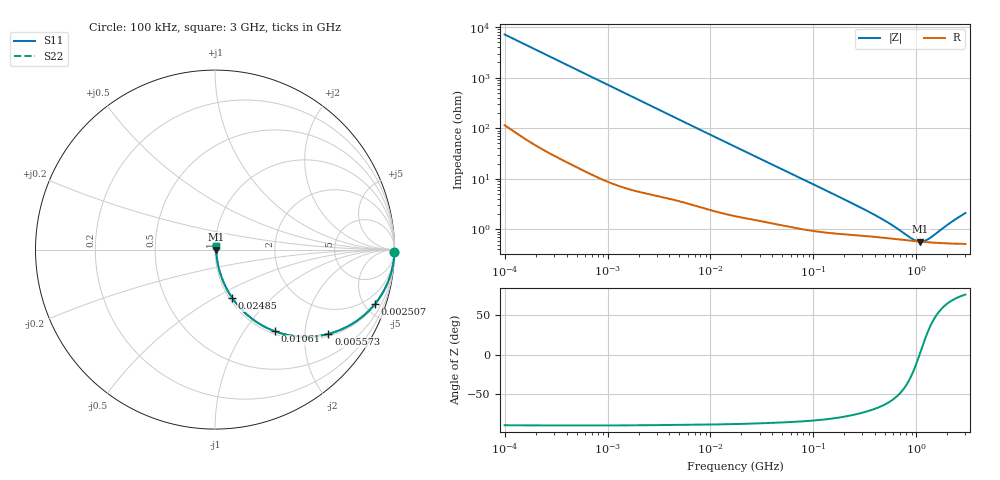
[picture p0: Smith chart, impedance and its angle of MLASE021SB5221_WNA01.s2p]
! MLASE021SB5221_WNA01  S-PARAMETER MODEL  ( Standard Model )
! Model Generated by TAIYO YUDEN Corporation (http://www.ty-top.com)
! Version 1.0
! TAIYO YUDEN Control No. 220901
! Copyright(c) 2022 TAIYO YUDEN CO.,LTD. All Rights Reserved.
! Product Description (link to TY-COMPAS)
! https://ds.yuden.co.jp/TYCOMPAS/or/detail?pn=MLASE021SB5221KWNA01&u=M
! Products Name : Multilayer Ceramic Capacitors
! Characteristics :
!  Capacitance : 220 [pF] , Rated Voltage : 16 [V] , TCC : X5R
!  Case Size : 0.25 x 0.125 / 0.0098 x 0.0049 [mm/inch] , Thickness : 0.125 / 0.0049 [mm/inch]
!  (Conditions: Temperature = 25 [degC] , DC Bias Voltage = 0 [V])
! External Node Assignments :
!  1  o---| |---o  2
! GND o---------o GND
! Frequency Range : 100kHz  -  3GHz  [ 401 STEP ]
# MHZ S RI R 50
! Freq[MHz].  S11 Real  S11 Imag  S21 Real  S21 Imag  S12 Real  S12 Imag  S22 Real  S22 Imag
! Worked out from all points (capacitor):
!   401 points, 100 kHz to 3 GHz, reference 50 ohm
!   read as one part in series: C = 222 pF near 105.3 kHz
!   lowest |Z| = 572 mohm at 1.098 GHz (marker M1)
!   series resonance near 1.076 GHz, so ESL is about 98 pH
!   S11 on the Smith chart (normalised r, x): 100 kHz: open; 2.507 MHz: 1.10, -5.81; 5.573 MHz: 1.07, -2.64; 10.61 MHz: 1.05, -1.40; 24.85 MHz: 1.03, -0.61; 3 GHz: 1.01, +0.04
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0.1  0.9996 -0.014  0.00042 0.014  0.00042 0.014  0.9996 -0.014
0.266273  0.9982 -0.0369  0.00181 0.0369  0.00181 0.0369  0.9982 -0.0369
0.562235  0.9931 -0.0772  0.0069 0.0772  0.0069 0.0772  0.9931 -0.0772
1.218153  0.9707 -0.1625  0.0293 0.1625  0.0293 0.1625  0.9707 -0.1625
2.506689  0.8901 -0.3043  0.1099 0.3043  0.1099 0.3043  0.8901 -0.3043
3.161081  0.8374 -0.3594  0.1626 0.3594  0.1626 0.3594  0.8374 -0.3594
4.197169  0.7481 -0.423  0.2519 0.423  0.2519 0.423  0.7481 -0.423
5.572849  0.6321 -0.4696  0.3679 0.4696  0.3679 0.4696  0.6321 -0.4696
7.592607  0.4868 -0.4855  0.5132 0.4855  0.5132 0.4855  0.4868 -0.4855
10.61445  0.3337 -0.4552  0.6663 0.4552  0.6663 0.4552  0.3337 -0.4552
17.7727  0.1609 -0.3466  0.8391 0.3466  0.8391 0.3466  0.1609 -0.3466
24.84619  0.0957 -0.2693  0.9043 0.2693  0.9043 0.2693  0.0957 -0.2693
47.32384  0.0365 -0.1534  0.9635 0.1534  0.9635 0.1534  0.0365 -0.1534
97.38194  0.0153 -0.0773  0.9847 0.0773  0.9847 0.0773  0.0153 -0.0773
310.5665  0.00792 -0.0235  0.9921 0.0235  0.9921 0.0235  0.00792 -0.0235
547.5153  0.00671 -0.0112  0.9933 0.0112  0.9933 0.0112  0.00671 -0.0112
916.7529  0.00588 -0.00257  0.9941 0.00257  0.9941 0.00257  0.00588 -0.00257
1097.999  0.00568 0.000328  0.9943 -0.000328  0.9943 -0.000328  0.00568 0.000328
1217.231  0.00558 0.00201  0.9944 -0.00201  0.9944 -0.00201  0.00558 0.00201
1349.411  0.00551 0.00373  0.9945 -0.00373  0.9945 -0.00373  0.00551 0.00373
2201.951  0.00538 0.0129  0.9946 -0.0129  0.9946 -0.0129  0.00538 0.0129
3000  0.00554 0.0202  0.9945 -0.0202  0.9945 -0.0202  0.00554 0.0202
